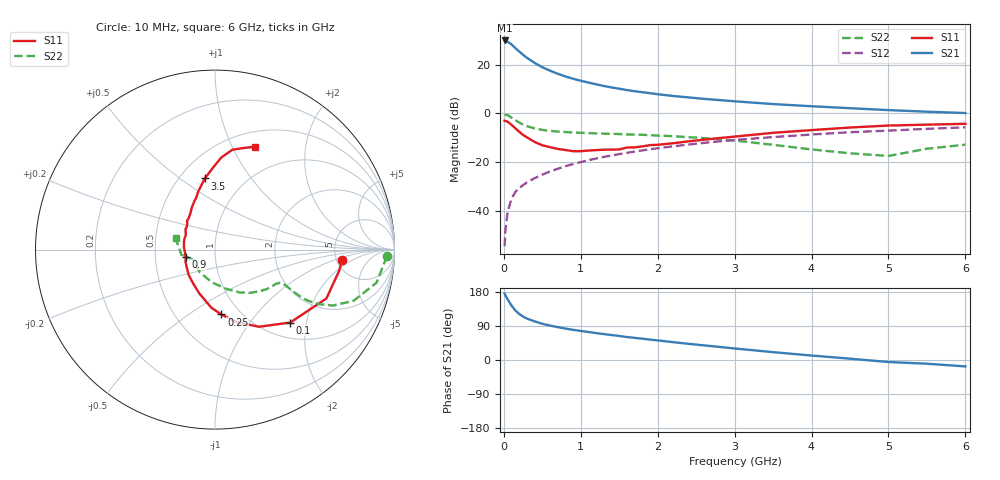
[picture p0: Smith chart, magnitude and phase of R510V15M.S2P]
! SIEMENS Small Signal Semiconductors
! BFR183
! Si NPN RF Bipolar Junction Transistor in SOT23
! VCE = 10 V  IC = 15 mA
! Common Emitter S-Parameters:  May  1996
# GHz  S  MA  R  50
!  f  S11  S21  S12  S22
! GHz  MAG  ANG  MAG  ANG  MAG  ANG  MAG  ANG
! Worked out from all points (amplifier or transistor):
!   36 points, 10 MHz to 6 GHz, reference 50 ohm
!   highest |S21| = 29.9 dB at 10 MHz (marker M1)
!   |S21| within 3 dB of that: start of sweep to 145.5 MHz
!   unconditionally stable (mu >= 1): 717.8 MHz to 2.638 GHz
!   at 250 MHz: K = 0.71, MSG = 26.7 dB, |S12| = -29.4 dB
!   at 1.4 GHz: K = 1.05, MAG = 12.6 dB, |S12| = -17.2 dB
!   at 6 GHz: K = 0.90, MSG = 2.9 dB, |S12| = -5.7 dB
!   S11 on the Smith chart (normalised r, x): 10 MHz: 5.54, -1.32; 100 MHz: 1.31, -1.62; 250 MHz: 0.82, -0.68; 900 MHz: 0.72, -0.06; 3.5 GHz: 0.66, +0.62; 6 GHz: 0.67, +1.23
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0.01  0.7086 -4.8  31.38 175.1  0.0019 79.7  0.9586 -2.2
0.02  0.7024 -9.5  30.66 171.0  0.004 78.7  0.9448 -4.8
0.05  0.6779 -23.7  29.56 159.9  0.0096 79.8  0.9186 -11.6
0.1  0.5837 -44.1  26.09 143.5  0.018 71.4  0.8227 -20.3
0.15  0.495 -60.3  21.87 130.6  0.0245 66.9  0.7268 -25.4
0.2  0.4227 -73.2  18.63 121.6  0.0296 65.9  0.6509 -27.8
0.25  0.3633 -84.4  15.95 114.5  0.0339 65.1  0.5897 -28.8
0.3  0.3242 -93.6  13.82 109.3  0.0386 65.9  0.5481 -28.9
0.4  0.26 -109.5  10.88 101.9  0.0471 66.5  0.4948 -28.2
0.5  0.2228 -123.7  8.88 95.6  0.0555 67.4  0.4602 -27.4
0.6  0.2037 -136.0  7.534 90.8  0.0646 67.8  0.439 -26.9
0.7  0.1873 -146.9  6.533 86.7  0.0732 68.4  0.4259 -26.8
0.9  0.1684 -166.8  5.144 79.7  0.092 67.9  0.4073 -27.1
1.1  0.1736 176.2  4.295 73.9  0.11 67.2  0.3952 -28.6
1.3  0.1806 161.7  3.659 68.4  0.1286 66.0  0.3854 -30.1
1.6  0.2002 145.2  3.015 60.6  0.1559 63.4  0.3713 -33.9
2.2  0.245 123.9  2.282 47.1  0.2119 57.9  0.3418 -43.0
3.5  0.4007 98.1  1.557 20.7  0.3278 42.4  0.2274 -74.0
4.5  0.5145 86.1  1.282 3.5  0.4128 30.3  0.1523 -123.5
5  0.5651 80.1  1.171 -5.3  0.4444 23.2  0.1345 -155.0
5.5  0.5893 74.0  1.086 -9.8  0.4836 19.1  0.1892 -171.2
6  0.6139 68.9  1.021 -16.9  0.5186 11.8  0.2287 164.0
